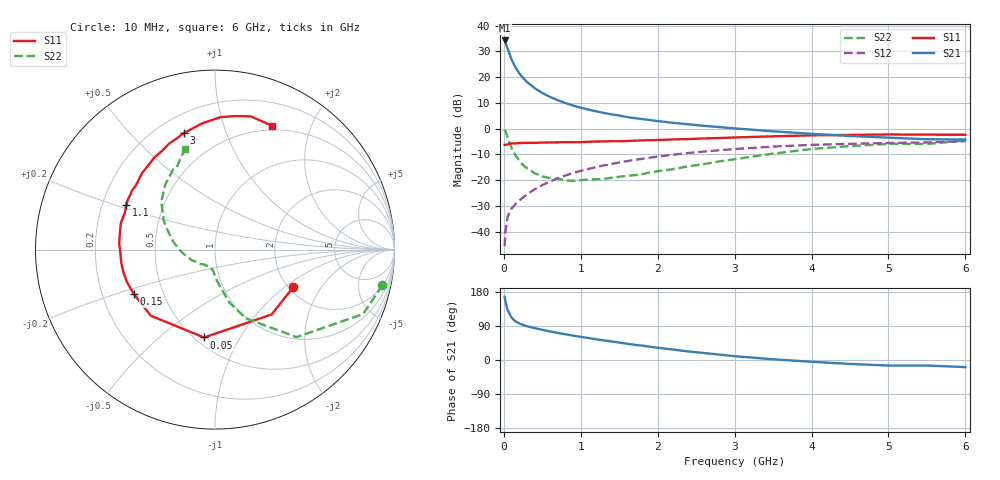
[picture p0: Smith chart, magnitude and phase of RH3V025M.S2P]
! SIEMENS Small Signal Semiconductors
! BFR106
! Si NPN RF Bipolar Junction Transistor in SOT23
! VCE = 3 V  IC = 25 mA
! Common Emitter S-Parameters:  August  1996
# GHz  S  MA  R  50
!  f  S11  S21  S12  S22
! GHz  MAG  ANG  MAG  ANG  MAG  ANG  MAG  ANG
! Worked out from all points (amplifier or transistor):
!   36 points, 10 MHz to 6 GHz, reference 50 ohm
!   highest |S21| = 34.2 dB at 10 MHz (marker M1)
!   |S21| within 3 dB of that: start of sweep to 46.76 MHz
!   unconditionally stable (mu >= 1): 325.8 MHz to 2.316 GHz; 5.383 GHz to end of sweep
!   at 250 MHz: K = 0.94, MSG = 23.2 dB, |S12| = -26.8 dB
!   at 1.4 GHz: K = 1.07, MAG = 8.1 dB, |S12| = -13.7 dB
!   at 6 GHz: K = 1.01, MAG = -0.1 dB, |S12| = -4.9 dB
!   S11 on the Smith chart (normalised r, x): 10 MHz: 2.11, -1.16; 50 MHz: 0.55, -0.72; 150 MHz: 0.34, -0.23; 1.1 GHz: 0.30, +0.22; 3 GHz: 0.30, +0.72; 6 GHz: 0.45, +1.47
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0.01  0.4834 -25.7  51.39 166.5  0.0052 81.9  0.9533 -12.0
0.02  0.4797 -48.9  48.08 155.5  0.0098 74.2  0.8998 -23.5
0.05  0.4933 -97.1  35.17 131.1  0.0198 58.7  0.6667 -47.0
0.1  0.5135 -134.2  22 112.0  0.0278 55.1  0.421 -65.7
0.15  0.5154 -151.3  15.45 102.2  0.034 55.9  0.3036 -75.1
0.2  0.5234 -160.2  11.9 96.7  0.04 58.6  0.2382 -79.1
0.25  0.5258 -166.7  9.578 92.3  0.0458 61.1  0.1944 -83.7
0.3  0.5271 -171.5  8.036 89.2  0.0526 63.0  0.1708 -86.8
0.4  0.5282 -178.6  6.101 84.1  0.0659 65.3  0.1363 -91.5
0.5  0.5347 176.4  4.903 79.6  0.0799 66.6  0.1173 -95.2
0.6  0.537 171.5  4.117 75.4  0.094 67.0  0.1094 -99.0
0.7  0.5406 167.6  3.562 71.4  0.1081 66.9  0.1046 -103.8
0.9  0.5426 160.3  2.799 64.4  0.137 65.6  0.0965 -111.7
1.1  0.5538 153.5  2.338 57.9  0.1646 63.8  0.1022 -120.5
1.3  0.5617 147.1  2.01 51.7  0.1926 61.4  0.1051 -129.4
1.6  0.5729 138.7  1.675 43.0  0.2333 57.5  0.1206 -142.4
2.2  0.6144 123.4  1.292 27.6  0.3107 48.8  0.1629 -166.7
3  0.6718 105.0  1.007 10.1  0.3999 36.4  0.2535 165.0
3.5  0.7066 95.9  0.885 1.9  0.447 28.7  0.3261 151.0
4.5  0.7533 81.0  0.717 -10.4  0.505 13.8  0.4565 127.3
5.5  0.7612 69.4  0.62 -14.7  0.5377 4.1  0.5025 115.5
6  0.7602 65.2  0.612 -18.7  0.567 -3.1  0.584 106.7
